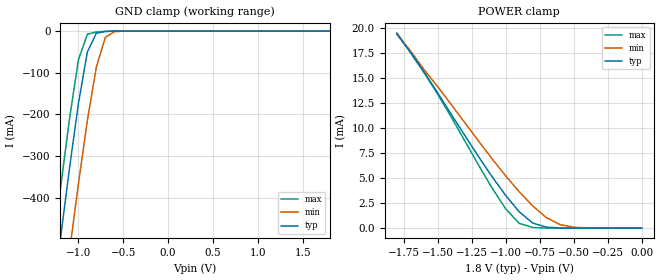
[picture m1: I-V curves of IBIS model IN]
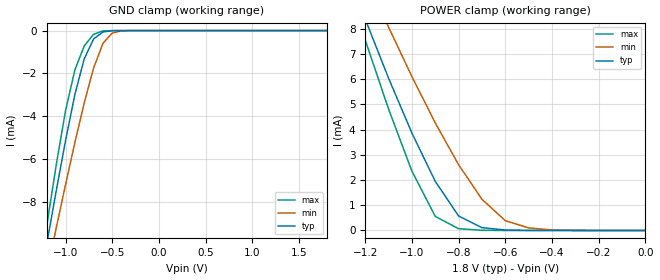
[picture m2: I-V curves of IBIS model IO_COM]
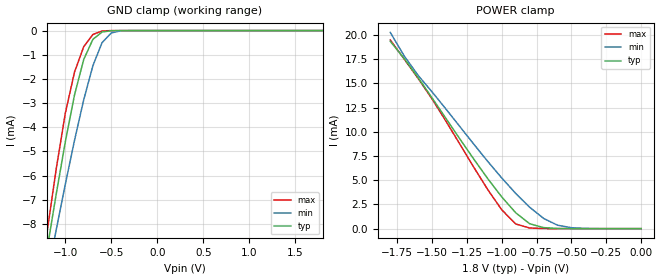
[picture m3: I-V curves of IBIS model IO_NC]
| (C) Copyright DIODES INCORPORATED
| DIODES CORPORATION
| IBIS Model of PI5A23157
| UQFN-10 (ZUA) Package
[IBIS Ver] 3.2
[Comment char] |_char
[File Name] pi5a23157_zua_18v.ibs
[File Rev] 1.0
[Source] File originated at Diodes Incorporated.
[Date] 28/11/24
[Disclaimer]
   All rights reserved
  DIODES Corporation hereby grants the user of
  this IBIS model a non-exclusive, nontransferable license to
  use this IBIS model under the following terms.
  This IBIS model is provided on an "AS IS" basis and Diodes
  makes absolutely no warranty with respect to the information
  contained herein. DIODES DISCLAIMS AND CUSTOMER WAIVES ALL
  WARRANTIES, EXPRESSED OR IMPLIED, INCLUDING WARRANTIES OF
  MERCHANTABILITY OR FITNESS FOR A PARTICULAR PURPOSE. The
  entire risk as to quality and performance is with the customer.
  Accordingly, in no event shall the company be liable for any
  damages, whether in contract or tort, including any lost
  profits or other incidental, consequential, exemplary, or
  punitive damages arising out of the use or application of the
  IBIS model provided in this package. Further, Diodes reserves
  the right to make changes without notice to any product herein
  to improve reliability, function, or design. Diodes does not
  convey any license under patent rights or any other intellectual
  property rights, including those of third parties.
  The user is granted this license only to use the IBIS model
  and is not granted rights to sell, load, rent, lease or license
  the IBIS model in whole or in part, or in modified form to anyone
  other than user. User may modify the IBIS model to suit its specific
  application but rights to derivative works and such modifications
  shall belong to Diodes.
  Diodes is not obligated to provide maintenance or support
  for the licensed IBIS model.
  Contact Diodes at ATTN: APPLICATION ENGINEERING / IBIS MODELS
  1545 Barber Lane Milpitas, CA 95035 USA.
[Component] PI5A23157
[Manufacturer] DIODES CORPORATION
[Package]
|   typ   min   max
R_pkg   50m   45m   55m
L_pkg   1.2n   1.08n   1.32n
C_pkg   0.35p   0.315p   0.385p
[Pin]   signal_name   model_name
1   IN1   IN
2   NO1   IO_NO
3   GND   GND
4   NO2   IO_NO
5   IN2   IN
6   COM2   IO_COM
7   NC2   IO_NC
8   VDD   POWER
9   NC1   IO_NC
10   COM1   IO_COM
[Series Switch Groups]
On   1 /   |NC1 to COM1
On   2 /   |NC2 to COM2
On   3 /   |NO1 to COM1
On   4 /   |NO2 to COM2
On   1 2 /
On   3 4 /
On   1 4 /
On   2 3 /
[Series Pin Mapping]   pin_2   model_name   function_table_group
9   10   SW_18   1
7   6   SW_18   2
2   10   SW_18   3
4   6   SW_18   4
[Model] SW_18
Model_type   Series_switch
Polarity   Non-Inverting
Enable  Active-High
C_comp   8.247pF   8.159pF   8.395pF
[Voltage Range]   1.8   1.65   1.95
[Temperature Range]   25   -40   125
[On]
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[off]
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| Models and submodels in the file (5): IN (Input), IO_COM (Terminator), IO_NC (Terminator), IO_NO (Terminator), SW_18 (Series_switch)
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[Model]   IN
Polarity   Non-Inverting
Model_type   Input
Vinl=0.54
Vinh=1.26
C_comp   1.924pF   1.914pF   1.943pF
[Voltage Range]   1.8   1.65   1.95
[Temperature Range]   25   -40   125
[GND Clamp Reference]   0   0   0
[POWER Clamp Reference]   1.8   1.65   1.95
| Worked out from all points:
|   GND clamp passes 1 mA (typ) near -0.69 V on its own axis
|   POWER clamp passes 1 mA (typ) near -0.84 V on its own axis
[GND_Clamp]
-1.8V     -1.57A     -1.768A    -1.454A
-1.3V     -672mA     -874.9mA   -551.1mA
-1.2V     -498.6mA   -701.3mA   -377.7mA
-1.1V     -330.7mA   -531.4mA   -212.2mA
-1V       -174.4mA   -367.4mA   -69.35mA
-900mV    -50.06mA   -214.6mA   -7.417mA
-800mV    -5.194mA   -86.41mA   -2.283mA
-700mV    -1.045mA   -15.38mA   -516.4uA
-600mV    -172uA     -1.514mA   -42.54uA
1.8V      65.92pA    854.3pA    64.8pA
[Power_Clamp]
|   X   TYP   MIN   MAX
-1.8V     19.33mA    19.4mA     19.47mA
-1.7V     17.55mA    17.67mA    17.5mA
-1.5V     13.49mA    14.11mA    13.37mA
-1.1V     5.146mA    6.927mA    4.014mA
-1V       3.269mA    5.225mA    1.939mA
-900mV    1.637mA    3.634mA    481.1uA
-800mV    504.8uA    2.208mA    68.25uA
-700mV    107.2uA    1.056mA    7.789uA
-600mV    18.47uA    353.6uA    572.5nA
-500mV    1.916uA    98.22uA    23.25nA
-400mV    132.7nA    19.45uA    1.282nA
0V        267.4pA    3.121nA    282.4pA
[Model]   IO_COM
Model_type   Terminator
C_comp   8.248pF   8.159pF   8.469pF
[Voltage Range]   1.8   1.65   1.95
[Temperature Range]   25   -40   125
[GND Clamp Reference]   0   0   0
[POWER Clamp Reference]   1.8   1.65   1.95
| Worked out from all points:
|   GND clamp passes 1 mA (typ) near -0.77 V on its own axis
|   POWER clamp passes 1 mA (typ) near -0.83 V on its own axis
[GND_Clamp]
-1.8V     -63.94mA   -661mA     -26.6mA
-1.3V     -12.44mA   -14.11mA   -11.98mA
-1.2V     -9.946mA   -11.35mA   -9.087mA
-1.1V     -7.493mA   -9.228mA   -6.28mA
-1V       -5.133mA   -7.194mA   -3.73mA
-900mV    -2.979mA   -5.229mA   -1.833mA
-800mV    -1.318mA   -3.377mA   -713.6uA
-700mV    -393.5uA   -1.751mA   -174.9uA
-600mV    -64.7uA    -597.4uA   -15.81uA
-500mV    -5.831uA   -111.9uA   -625.9nA
-400mV    -349nA     -12.01uA   -14.65nA
1.8V      353.3pA    73.79nA    201.1pA
[Power_Clamp]
-1.8V     24.84mA    24.99mA    26.68mA
-1.3V     10.86mA    12.34mA    10.47mA
-1.2V     8.386mA    10.15mA    7.557mA
-1.1V     6.04mA     8.069mA    4.815mA
-1V       3.863mA    6.103mA    2.352mA
-900mV    1.946mA    4.266mA    557.1uA
-800mV    573.4uA    2.606mA    69.97uA
-700mV    110.6uA    1.235mA    7.898uA
-600mV    18.78uA    388.2uA    579.2nA
-500mV    1.94uA     101.5uA    23.57nA
-400mV    134.4nA    19.83uA    1.3nA
0V        354.2pA    3.32nA     368.5pA
[Model]   IO_NC
Model_type   Terminator
C_comp   3.078pF   3.046pF   3.195pF
[Voltage Range]   1.8   1.65   1.95
[Temperature Range]   25   -40   125
[GND Clamp Reference]   0   0   0
[POWER Clamp Reference]   1.8   1.65   1.95
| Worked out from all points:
|   GND clamp passes 1 mA (typ) near -0.78 V on its own axis
|   POWER clamp passes 1 mA (typ) near -0.84 V on its own axis
[GND_Clamp]
-1.8V     -43.97mA   -353.4mA   -25.26mA
-1.2V     -9.098mA   -10.25mA   -8.383mA
-1.1V     -6.79mA    -8.263mA   -5.753mA
-1V       -4.605mA   -6.359mA   -3.421mA
-900mV    -2.662mA   -4.541mA   -1.717mA
-800mV    -1.198mA   -2.865mA   -669.7uA
-700mV    -360.7uA   -1.451mA   -161.7uA
-600mV    -59.18uA   -497.6uA   -14.42uA
-500mV    -5.324uA   -97.48uA   -563nA
-400mV    -315.9nA   -10.75uA   -13.07nA
1.8V      267.8pA    72.57nA    181.9pA
[Power_Clamp]
-1.8V     19.33mA    20.25mA    19.47mA
-1.7V     17.55mA    17.82mA    17.5mA
-1.6V     15.58mA    15.81mA    15.5mA
-1.4V     11.36mA    12.33mA    11.08mA
-1.1V     5.146mA    6.927mA    4.014mA
-1V       3.269mA    5.225mA    1.939mA
-900mV    1.637mA    3.634mA    481.1uA
-800mV    504.8uA    2.208mA    68.25uA
-700mV    107.2uA    1.056mA    7.789uA
-600mV    18.47uA    353.6uA    572.5nA
-400mV    132.7nA    19.45uA    1.282nA
0V        267.4pA    3.121nA    282.4pA
